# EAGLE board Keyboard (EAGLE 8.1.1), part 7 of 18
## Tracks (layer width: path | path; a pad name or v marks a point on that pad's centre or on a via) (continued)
S$6559 (continued)
  Bottom 0: 112.13,25.25 111.81,25.4
S$6560
  Bottom 0: 111.81,25.4 111.47,25.46
S$6561
  Bottom 0: 111.47,25.46 111.12,25.44
S$6562
  Bottom 0: 111.12,25.44 110.82,25.34
S$6563
  Bottom 0: 110.82,25.34 111.79,26.32
S$6564
  Bottom 0: 111.79,26.32 111.85,26.38
S$6565
  Bottom 0: 111.85,26.38 111.9,26.46
S$6566
  Bottom 0: 111.9,26.46 111.94,26.54
S$6567
  Bottom 0: 111.94,26.54 111.96,26.63
S$6568
  Bottom 0: 111.96,26.63 111.96,26.72
S$6569
  Bottom 0: 111.96,26.72 111.96,33.9
S$6570
  Bottom 0: 111.96,33.9 112.2,34.07
S$6571
  Bottom 0: 112.2,34.07 112.41,34.32
S$6572
  Bottom 0: 112.41,34.32 112.54,34.62
S$6573
  Bottom 0: 112.54,34.62 112.58,34.94
S$6574
  Bottom 0: 112.58,34.94 112.54,35.26
S$6575
  Bottom 0: 112.54,35.26 112.41,35.56
S$6576
  Bottom 0: 112.41,35.56 112.2,35.82
S$6577
  Bottom 0: 112.2,35.82 112.03,35.94
S$6578
  Bottom 0: 112.03,35.94 112.63,35.94
S$6579
  Bottom 0: 112.63,35.94 112.7,35.94
S$6580
  Bottom 0: 112.7,35.94 112.76,35.96
S$6581
  Bottom 0: 112.76,35.96 112.82,35.98
S$6582
  Bottom 0: 112.82,35.98 112.88,36.02
S$6583
  Bottom 0: 112.88,36.02 112.94,36.06
S$6584
  Bottom 0: 112.94,36.06 117.28,40.4
S$6585
  Bottom 0: 117.28,40.4 117.32,40.46
S$6586
  Bottom 0: 117.32,40.46 117.36,40.52
S$6587
  Bottom 0: 117.36,40.52 117.39,40.58
S$6588
  Bottom 0: 117.39,40.58 117.4,40.65
S$6589
  Bottom 0: 117.4,40.65 117.41,40.72
S$6590
  Bottom 0: 117.41,40.72 117.41,41.83
S$6591
  Bottom 0: 117.41,41.83 122.58,47
S$6592
  Bottom 0: 122.58,47 122.63,47.05
S$6593
  Bottom 0: 122.63,47.05 122.67,47.11
S$6594
  Bottom 0: 122.67,47.11 122.69,47.17
S$6595
  Bottom 0: 122.69,47.17 122.71,47.24
S$6596
  Bottom 0: 122.71,47.24 122.72,47.31
S$6597
  Bottom 0: 122.72,47.31 122.72,56.03
S$6598
  Bottom 0: 122.72,56.03 122.71,56.1
S$6599
  Bottom 0: 122.71,56.1 122.69,56.17
S$6600
  Bottom 0: 122.69,56.17 122.67,56.23
S$6601
  Bottom 0: 122.67,56.23 122.63,56.29
S$6602
  Bottom 0: 122.63,56.29 122.59,56.34
S$6603
  Bottom 0: 122.59,56.34 117.39,61.54
S$6604
  Bottom 0: 117.39,61.54 117.49,61.82
S$6605
  Bottom 0: 117.49,61.82 117.54,62.17
S$6606
  Bottom 0: 117.54,62.17 117.49,62.51
S$6607
  Bottom 0: 117.49,62.51 117.37,62.84
S$6608
  Bottom 0: 117.37,62.84 117.16,63.12
S$6609
  Bottom 0: 117.16,63.12 116.89,63.34
S$6610
  Bottom 0: 116.89,63.34 116.58,63.49
S$6611
  Bottom 0: 116.58,63.49 116.58,64.42
S$6612
  Bottom 0: 116.58,64.42 116.58,64.49
S$6613
  Bottom 0: 116.58,64.49 116.56,64.56
S$6614
  Bottom 0: 116.56,64.56 116.53,64.62
S$6615
  Bottom 0: 116.53,64.62 116.5,64.68
S$6616
  Bottom 0: 116.5,64.68 116.45,64.74
S$6617
  Bottom 0: 116.45,64.74 113.01,68.18
S$6618
  Bottom 0: 113.01,68.18 112.96,68.21
S$6619
  Bottom 0: 112.96,68.21 112.89,68.26
S$6620
  Bottom 0: 112.89,68.26 112.83,68.28
S$6621
  Bottom 0: 112.83,68.28 112.77,68.3
S$6622
  Bottom 0: 112.77,68.3 112.7,68.3
S$6623
  Bottom 0: 112.7,68.3 110.8,68.3
S$6624
  Bottom 0: 110.8,68.3 110.46,68.64
S$6625
  Bottom 0: 110.46,68.64 111.95,68.64
S$6626
  Bottom 0: 111.95,68.64 112.02,68.65
S$6627
  Bottom 0: 112.02,68.65 112.1,68.69
S$6628
  Bottom 0: 112.1,68.69 112.15,68.75
S$6629
  Bottom 0: 112.15,68.75 112.19,68.82
S$6630
  Bottom 0: 112.19,68.82 112.2,68.9
S$6631
  Bottom 0: 112.2,68.9 112.2,70.67
S$6632
  Bottom 0: 112.2,70.67 112.19,70.75
S$6633
  Bottom 0: 112.19,70.75 112.15,70.82
S$6634
  Bottom 0: 112.15,70.82 112.1,70.88
S$6635
  Bottom 0: 112.1,70.88 112.02,70.92
S$6636
  Bottom 0: 112.02,70.92 111.95,70.93
S$6637
  Bottom 0: 111.95,70.93 111.5,70.93
S$6638
  Bottom 0: 111.5,70.93 111.5,71.06
S$6639
  Bottom 0: 111.5,71.06 111.44,71.28
S$6640
  Bottom 0: 111.44,71.28 111.28,71.44
S$6641
  Bottom 0: 111.28,71.44 111.06,71.5
S$6642
  Bottom 0: 111.06,71.5 110.71,71.5
S$6643
  Bottom 0: 110.71,71.5 109.62,72.58
S$6644
  Bottom 0: 109.62,72.58 109.68,72.72
S$6645
  Bottom 0: 109.68,72.72 109.72,73.04
S$6646
  Bottom 0: 109.72,73.04 109.68,73.36
S$6647
  Bottom 0: 109.68,73.36 109.55,73.66
S$6648
  Bottom 0: 109.55,73.66 109.34,73.92
S$6649
  Bottom 0: 109.34,73.92 109.08,74.11
S$6650
  Bottom 0: 109.08,74.11 108.78,74.21
S$6651
  Bottom 0: 108.78,74.21 108.45,74.23
S$6652
  Bottom 0: 108.45,74.23 108.13,74.17
S$6653
  Bottom 0: 108.13,74.17 107.84,74.02
S$6654
  Bottom 0: 107.84,74.02 107.61,73.8
S$6655
  Bottom 0: 107.61,73.8 107.43,73.52
S$6656
  Bottom 0: 107.43,73.52 107.35,73.2
S$6657
  Bottom 0: 107.35,73.2 107.35,72.88
S$6658
  Bottom 0: 107.35,72.88 107.43,72.56
S$6659
  Bottom 0: 107.43,72.56 107.61,72.29
S$6660
  Bottom 0: 107.61,72.29 107.84,72.07
S$6661
  Bottom 0: 107.84,72.07 108.13,71.92
S$6662
  Bottom 0: 108.13,71.92 108.45,71.85
S$6663
  Bottom 0: 108.45,71.85 108.78,71.87
S$6664
  Bottom 0: 108.78,71.87 109,71.95
S$6665
  Bottom 0: 109,71.95 110.06,70.9
S$6666
  Bottom 0: 110.06,70.9 110.02,70.88
S$6667
  Bottom 0: 110.02,70.88 109.97,70.82
S$6668
  Bottom 0: 109.97,70.82 109.93,70.75
S$6669
  Bottom 0: 109.93,70.75 109.92,70.67
S$6670
  Bottom 0: 109.92,70.67 109.92,69.19
S$6671
  Bottom 0: 109.92,69.19 106.29,72.82
S$6672
  Bottom 0: 106.29,72.82 106.33,73.03
S$6673
  Bottom 0: 106.33,73.03 106.28,73.28
S$6674
  Bottom 0: 106.28,73.28 106.15,73.49
S$6675
  Bottom 0: 106.15,73.49 105.95,73.64
S$6676
  Bottom 0: 105.95,73.64 105.72,73.7
S$6677
  Bottom 0: 105.72,73.7 106.29,74.28
S$6678
  Bottom 0: 106.29,74.28 106.55,74.23
S$6679
  Bottom 0: 106.55,74.23 106.87,74.24
S$6680
  Bottom 0: 106.87,74.24 107.17,74.35
S$6681
  Bottom 0: 107.17,74.35 107.44,74.54
S$6682
  Bottom 0: 107.44,74.54 107.64,74.8
S$6683
  Bottom 0: 107.64,74.8 107.77,75.09
S$6684
  Bottom 0: 107.77,75.09 107.82,75.42
S$6685
  Bottom 0: 107.82,75.42 107.77,75.73
S$6686
  Bottom 0: 107.77,75.73 107.64,76.03
S$6687
  Bottom 0: 107.64,76.03 107.44,76.29
S$6688
  Bottom 0: 107.44,76.29 108.3,76.29
S$6689
  Bottom 0: 108.3,76.29 113.67,70.92
S$6690
  Bottom 0: 113.67,70.92 113.44,70.92
S$6691
  Bottom 0: 113.44,70.92 113.13,70.83
S$6692
  Bottom 0: 113.13,70.83 112.85,70.65
S$6693
  Bottom 0: 112.85,70.65 112.64,70.41
S$6694
  Bottom 0: 112.64,70.41 112.5,70.11
S$6695
  Bottom 0: 112.5,70.11 112.46,69.79
S$6696
  Bottom 0: 112.46,69.79 112.5,69.47
S$6697
  Bottom 0: 112.5,69.47 112.64,69.16
S$6698
  Bottom 0: 112.64,69.16 112.85,68.92
S$6699
  Bottom 0: 112.85,68.92 113.13,68.75
S$6700
  Bottom 0: 113.13,68.75 113.44,68.65
S$6701
  Bottom 0: 113.44,68.65 113.76,68.65
S$6702
  Bottom 0: 113.76,68.65 114.07,68.75
S$6703
  Bottom 0: 114.07,68.75 114.35,68.92
S$6704
  Bottom 0: 114.35,68.92 114.56,69.16
S$6705
  Bottom 0: 114.56,69.16 114.7,69.47
S$6706
  Bottom 0: 114.7,69.47 114.75,69.79
S$6707
  Bottom 0: 114.75,69.79 114.73,69.85
S$6708
  Bottom 0: 114.73,69.85 123.81,60.77
S$6709
  Bottom 0: 123.81,60.77 123.81,41.6
S$6710
  Bottom 0: 123.81,41.6 113.64,31.45
S$6711
  Bottom 0: 113.64,31.45 113.61,31.39
S$6712
  Bottom 0: 113.61,31.39 113.57,31.33
S$6713
  Bottom 0: 113.57,31.33 113.54,31.27
S$6714
  Bottom 0: 113.54,31.27 113.53,31.2
S$6715
  Bottom 0: 113.53,31.2 113.52,31.13
S$6716
  Bottom 0: 113.52,31.13 113.52,23.41
S$6717
  Bottom 0: 113.52,23.41 113.38,23.26
S$6718
  Bottom 0: 113.38,23.26 113.29,23.02
S$6719
  Bottom 0: 113.29,23.02 113.29,22.77
S$6720
  Bottom 0: 113.29,22.77 113.38,22.54
S$6721
  Bottom 0: 113.38,22.54 113.55,22.35
S$6722
  Bottom 0: 113.55,22.35 113.77,22.24
S$6723
  Bottom 0: 113.77,22.24 114.02,22.22
S$6724
  Bottom 0: 114.02,22.22 114.27,22.28
S$6725
  Bottom 0: 114.27,22.28 114.47,22.44
S$6726
  Bottom 0: 114.47,22.44 114.6,22.65
S$6727
  Bottom 0: 114.6,22.65 114.65,22.9
S$6728
  Bottom 0: 114.65,22.9 114.6,23.15
S$6729
  Bottom 0: 114.6,23.15 114.47,23.36
S$6730
  Bottom 0: 114.47,23.36 114.4,23.41
S$6731
  Bottom 0: 114.4,23.41 114.4,30.95
S$6732
  Bottom 0: 114.4,30.95 124.56,41.1
S$6733
  Bottom 0: 124.56,41.1 124.61,41.16
S$6734
  Bottom 0: 124.61,41.16 124.64,41.22
S$6735
  Bottom 0: 124.64,41.22 124.67,41.28
S$6736
  Bottom 0: 124.67,41.28 124.69,41.35
S$6737
  Bottom 0: 124.69,41.35 124.69,41.42
S$6738
  Bottom 0: 124.69,41.42 124.69,57.56
S$6739
  Bottom 0: 124.69,57.56 131.03,57.56
S$6740
  Bottom 0: 131.03,57.56 131.1,57.56
S$6741
  Bottom 0: 131.1,57.56 131.16,57.58
S$6742
  Bottom 0: 131.16,57.58 131.22,57.6
S$6743
  Bottom 0: 131.22,57.6 131.28,57.65
S$6744
  Bottom 0: 131.28,57.65 131.34,57.69
S$6745
  Bottom 0: 131.34,57.69 134.57,60.92
S$6746
  Bottom 0: 134.57,60.92 134.6,60.9
S$6747
  Bottom 0: 134.6,60.9 134.93,60.8
S$6748
  Bottom 0: 134.93,60.8 135.28,60.77
S$6749
  Bottom 0: 135.28,60.77 135.62,60.84
S$6750
  Bottom 0: 135.62,60.84 135.94,60.99
S$6751
  Bottom 0: 135.94,60.99 136.21,61.21
S$6752
  Bottom 0: 136.21,61.21 136.42,61.5
S$6753
  Bottom 0: 136.42,61.5 136.54,61.82
S$6754
  Bottom 0: 136.54,61.82 136.59,62.17
S$6755
  Bottom 0: 136.59,62.17 136.54,62.51
S$6756
  Bottom 0: 136.54,62.51 136.42,62.84
S$6757
  Bottom 0: 136.42,62.84 136.21,63.12
S$6758
  Bottom 0: 136.21,63.12 135.94,63.34
S$6759
  Bottom 0: 135.94,63.34 135.62,63.5
S$6760
  Bottom 0: 135.62,63.5 135.28,63.56
S$6761
  Bottom 0: 135.28,63.56 134.93,63.54
S$6762
  Bottom 0: 134.93,63.54 134.6,63.43
S$6763
  Bottom 0: 134.6,63.43 134.3,63.24
S$6764
  Bottom 0: 134.3,63.24 134.06,62.99
S$6765
  Bottom 0: 134.06,62.99 133.89,62.68
S$6766
  Bottom 0: 133.89,62.68 133.81,62.34
S$6767
  Bottom 0: 133.81,62.34 133.81,61.99
S$6768
  Bottom 0: 133.81,61.99 133.89,61.65
S$6769
  Bottom 0: 133.89,61.65 133.95,61.55
S$6770
  Bottom 0: 133.95,61.55 130.84,58.44
S$6771
  Bottom 0: 130.84,58.44 129.58,58.44
S$6772
  Bottom 0: 129.58,58.44 129.59,58.45
S$6773
  Bottom 0: 129.59,58.45 129.86,58.67
S$6774
  Bottom 0: 129.86,58.67 130.07,58.96
S$6775
  Bottom 0: 130.07,58.96 130.19,59.28
S$6776
  Bottom 0: 130.19,59.28 130.24,59.63
S$6777
  Bottom 0: 130.24,59.63 130.19,59.97
S$6778
  Bottom 0: 130.19,59.97 130.07,60.3
S$6779
  Bottom 0: 130.07,60.3 129.86,60.58
S$6780
  Bottom 0: 129.86,60.58 129.59,60.8
S$6781
  Bottom 0: 129.59,60.8 129.27,60.96
S$6782
  Bottom 0: 129.27,60.96 128.93,61.02
S$6783
  Bottom 0: 128.93,61.02 128.58,61
S$6784
  Bottom 0: 128.58,61 128.25,60.89
S$6785
  Bottom 0: 128.25,60.89 127.95,60.7
S$6786
  Bottom 0: 127.95,60.7 127.71,60.45
S$6787
  Bottom 0: 127.71,60.45 127.54,60.14
S$6788
  Bottom 0: 127.54,60.14 127.45,59.8
S$6789
  Bottom 0: 127.45,59.8 127.45,59.45
S$6790
  Bottom 0: 127.45,59.45 127.54,59.11
S$6791
  Bottom 0: 127.54,59.11 127.71,58.8
S$6792
  Bottom 0: 127.71,58.8 127.95,58.55
S$6793
  Bottom 0: 127.95,58.55 128.12,58.44
S$6794
  Bottom 0: 128.12,58.44 124.69,58.44
S$6795
  Bottom 0: 124.69,58.44 124.69,60.96
S$6796
  Bottom 0: 124.69,60.96 124.69,61.03
S$6797
  Bottom 0: 124.69,61.03 124.67,61.1
S$6798
  Bottom 0: 124.67,61.1 124.64,61.16
S$6799
  Bottom 0: 124.64,61.16 124.61,61.22
S$6800
  Bottom 0: 124.61,61.22 124.56,61.28
S$6801
  Bottom 0: 124.56,61.28 108.8,77.05
S$6802
  Bottom 0: 108.8,77.05 108.69,77.13
S$6803
  Bottom 0: 108.69,77.13 108.62,77.15
S$6804
  Bottom 0: 108.62,77.15 108.56,77.17
S$6805
  Bottom 0: 108.56,77.17 108.49,77.17
S$6806
  Bottom 0: 108.49,77.17 104.84,77.17
S$6807
  Bottom 0: 104.84,77.17 104.77,77.17
S$6808
  Bottom 0: 104.77,77.17 104.71,77.15
S$6809
  Bottom 0: 104.71,77.15 104.64,77.12
S$6810
  Bottom 0: 104.64,77.12 104.58,77.09
S$6811
  Bottom 0: 104.58,77.09 104.53,77.04
S$6812
  Bottom 0: 104.53,77.04 102.04,74.55
S$6813
  Bottom 0: 102.04,74.55 99.83,74.55
S$6814
  Bottom 0: 99.83,74.55 100.03,74.8
S$6815
  Bottom 0: 100.03,74.8 100.15,75.09
S$6816
  Bottom 0: 100.15,75.09 100.2,75.42
S$6817
  Bottom 0: 100.2,75.42 100.15,75.73
S$6818
  Bottom 0: 100.15,75.73 100.03,76.03
S$6819
  Bottom 0: 100.03,76.03 99.82,76.29
S$6820
  Bottom 0: 99.82,76.29 99.56,76.48
S$6821
  Bottom 0: 99.56,76.48 99.25,76.58
S$6822
  Bottom 0: 99.25,76.58 98.95,76.6
S$6823
  Bottom 0: 98.95,76.6 98.95,78.22
S$6824
  Bottom 0: 98.95,78.22 98.97,78.16
S$6825
  Bottom 0: 98.97,78.16 99.14,77.85
S$6826
  Bottom 0: 99.14,77.85 99.38,77.6
S$6827
  Bottom 0: 99.38,77.6 99.67,77.41
S$6828
  Bottom 0: 99.67,77.41 100,77.31
S$6829
  Bottom 0: 100,77.31 100.35,77.28
S$6830
  Bottom 0: 100.35,77.28 100.7,77.35
S$6831
  Bottom 0: 100.7,77.35 101.01,77.5
S$6832
  Bottom 0: 101.01,77.5 101.28,77.72
S$6833
  Bottom 0: 101.28,77.72 101.49,78.01
S$6834
  Bottom 0: 101.49,78.01 101.62,78.33
S$6835
  Bottom 0: 101.62,78.33 101.66,78.68
S$6836
  Bottom 0: 101.66,78.68 101.62,79.02
S$6837
  Bottom 0: 101.62,79.02 101.49,79.35
S$6838
  Bottom 0: 101.49,79.35 101.28,79.63
S$6839
  Bottom 0: 101.28,79.63 101.01,79.86
S$6840
  Bottom 0: 101.01,79.86 100.7,80.01
S$6841
  Bottom 0: 100.7,80.01 100.35,80.07
S$6842
  Bottom 0: 100.35,80.07 100,80.05
S$6843
  Bottom 0: 100,80.05 99.67,79.94
S$6844
  Bottom 0: 99.67,79.94 99.38,79.75
S$6845
  Bottom 0: 99.38,79.75 99.14,79.5
S$6846
  Bottom 0: 99.14,79.5 98.97,79.19
S$6847
  Bottom 0: 98.97,79.19 98.95,79.13
S$6848
  Bottom 0: 98.95,79.13 98.95,84.36
S$6849
  Bottom 0: 98.95,84.36 101.85,87.25
S$6850
  Bottom 0: 101.85,87.25 101.88,87.31
S$6851
  Bottom 0: 101.88,87.31 101.92,87.35
S$6852
  Bottom 0: 101.92,87.35 101.93,87.39
S$6853
  Bottom 0: 101.93,87.39 101.96,87.45
S$6854
  Bottom 0: 101.96,87.45 101.96,87.51
S$6855
  Bottom 0: 101.96,87.51 101.98,87.57
S$6856
  Bottom 0: 101.98,87.57 101.98,87.69
S$6857
  Bottom 0: 101.98,87.69 102.42,87.69
S$6858
  Bottom 0: 102.42,87.69 102.5,87.7
S$6859
  Bottom 0: 102.5,87.7 102.57,87.74
S$6860
  Bottom 0: 102.57,87.74 102.63,87.8
S$6861
  Bottom 0: 102.63,87.8 102.67,87.87
S$6862
  Bottom 0: 102.67,87.87 102.68,87.95
S$6863
  Bottom 0: 102.68,87.95 102.68,89.65
S$6864
  Bottom 0: 102.68,89.65 103.29,89.65
S$6865
  Bottom 0: 103.29,89.65 103.12,89.46
S$6866
  Bottom 0: 103.12,89.46 102.98,89.16
S$6867
  Bottom 0: 102.98,89.16 102.93,88.84
S$6868
  Bottom 0: 102.93,88.84 102.98,88.52
S$6869
  Bottom 0: 102.98,88.52 103.12,88.22
S$6870
  Bottom 0: 103.12,88.22 103.33,87.97
S$6871
  Bottom 0: 103.33,87.97 103.6,87.8
S$6872
  Bottom 0: 103.6,87.8 103.91,87.7
S$6873
  Bottom 0: 103.91,87.7 104.24,87.7
S$6874
  Bottom 0: 104.24,87.7 104.55,87.8
S$6875
  Bottom 0: 104.55,87.8 104.82,87.97
S$6876
  Bottom 0: 104.82,87.97 105.04,88.22
S$6877
  Bottom 0: 105.04,88.22 105.17,88.52
S$6878
  Bottom 0: 105.17,88.52 105.22,88.84
S$6879
  Bottom 0: 105.22,88.84 105.17,89.16
S$6880
  Bottom 0: 105.17,89.16 105.04,89.46
S$6881
  Bottom 0: 105.04,89.46 104.86,89.65
S$6882
  Bottom 0: 104.86,89.65 119.44,89.65
S$6883
  Bottom 0: 119.44,89.65 119.44,87.95
S$6884
  Bottom 0: 119.44,87.95 119.45,87.87
S$6885
  Bottom 0: 119.45,87.87 119.49,87.8
S$6886
  Bottom 0: 119.49,87.8 119.55,87.74
S$6887
  Bottom 0: 119.55,87.74 119.62,87.7
S$6888
  Bottom 0: 119.62,87.7 119.7,87.69
S$6889
  Bottom 0: 119.7,87.69 120.09,87.69
S$6890
  Bottom 0: 120.09,87.69 117.43,85.04
S$6891
  Bottom 0: 117.43,85.04 117.39,84.99
S$6892
  Bottom 0: 117.39,84.99 117.35,84.93
S$6893
  Bottom 0: 117.35,84.93 117.32,84.86
S$6894
  Bottom 0: 117.32,84.86 117.31,84.8
S$6895
  Bottom 0: 117.31,84.8 117.3,84.73
S$6896
  Bottom 0: 117.3,84.73 117.3,76.33
S$6897
  Bottom 0: 117.3,76.33 117.13,76.17
S$6898
  Bottom 0: 117.13,76.17 116.96,75.89
S$6899
  Bottom 0: 116.96,75.89 116.87,75.58
S$6900
  Bottom 0: 116.87,75.58 116.87,75.26
S$6901
  Bottom 0: 116.87,75.26 116.96,74.94
S$6902
  Bottom 0: 116.96,74.94 117.03,74.83
S$6903
  Bottom 0: 117.03,74.83 114.25,77.61
S$6904
  Bottom 0: 114.25,77.61 114.2,77.64
S$6905
  Bottom 0: 114.2,77.64 114.14,77.69
S$6906
  Bottom 0: 114.14,77.69 114.07,77.71
S$6907
  Bottom 0: 114.07,77.71 114.01,77.73
S$6908
  Bottom 0: 114.01,77.73 113.94,77.73
S$6909
  Bottom 0: 113.94,77.73 110.73,77.73
S$6910
  Bottom 0: 110.73,77.73 107.86,80.6
S$6911
  Bottom 0: 107.86,80.6 107.97,80.87
S$6912
  Bottom 0: 107.97,80.87 108.01,81.22
S$6913
  Bottom 0: 108.01,81.22 107.97,81.56
S$6914
  Bottom 0: 107.97,81.56 107.84,81.89
S$6915
  Bottom 0: 107.84,81.89 107.63,82.17
S$6916
  Bottom 0: 107.63,82.17 107.36,82.39
S$6917
  Bottom 0: 107.36,82.39 107.05,82.55
S$6918
  Bottom 0: 107.05,82.55 106.7,82.61
S$6919
  Bottom 0: 106.7,82.61 106.35,82.59
S$6920
  Bottom 0: 106.35,82.59 106.02,82.48
S$6921
  Bottom 0: 106.02,82.48 105.73,82.29
S$6922
  Bottom 0: 105.73,82.29 105.49,82.04
S$6923
  Bottom 0: 105.49,82.04 105.32,81.73
S$6924
  Bottom 0: 105.32,81.73 105.23,81.39
S$6925
  Bottom 0: 105.23,81.39 105.23,81.04
S$6926
  Bottom 0: 105.23,81.04 105.32,80.7
S$6927
  Bottom 0: 105.32,80.7 105.49,80.39
S$6928
  Bottom 0: 105.49,80.39 105.73,80.14
S$6929
  Bottom 0: 105.73,80.14 106.02,79.95
S$6930
  Bottom 0: 106.02,79.95 106.35,79.84
S$6931
  Bottom 0: 106.35,79.84 106.7,79.83
S$6932
  Bottom 0: 106.7,79.83 107.05,79.89
S$6933
  Bottom 0: 107.05,79.89 107.23,79.97
S$6934
  Bottom 0: 107.23,79.97 110.23,76.97
S$6935
  Bottom 0: 110.23,76.97 110.28,76.93
S$6936
  Bottom 0: 110.28,76.93 110.34,76.89
S$6937
  Bottom 0: 110.34,76.89 110.4,76.87
S$6938
  Bottom 0: 110.4,76.87 110.47,76.85
S$6939
  Bottom 0: 110.47,76.85 110.54,76.85
S$6940
  Bottom 0: 110.54,76.85 113.75,76.85
S$6941
  Bottom 0: 113.75,76.85 116.39,74.21
S$6942
  Bottom 0: 116.39,74.21 116.07,74.23
S$6943
  Bottom 0: 116.07,74.23 115.75,74.17
S$6944
  Bottom 0: 115.75,74.17 115.46,74.02
S$6945
  Bottom 0: 115.46,74.02 115.23,73.8
S$6946
  Bottom 0: 115.23,73.8 115.05,73.52
S$6947
  Bottom 0: 115.05,73.52 114.97,73.2
S$6948
  Bottom 0: 114.97,73.2 114.97,72.88
S$6949
  Bottom 0: 114.97,72.88 115.05,72.56
S$6950
  Bottom 0: 115.05,72.56 115.23,72.29
S$6951
  Bottom 0: 115.23,72.29 115.46,72.07
S$6952
  Bottom 0: 115.46,72.07 115.75,71.92
S$6953
  Bottom 0: 115.75,71.92 116.07,71.85
S$6954
  Bottom 0: 116.07,71.85 116.39,71.87
S$6955
  Bottom 0: 116.39,71.87 116.7,71.98
S$6956
  Bottom 0: 116.7,71.98 116.96,72.17
S$6957
  Bottom 0: 116.96,72.17 117.17,72.42
S$6958
  Bottom 0: 117.17,72.42 117.19,72.47
S$6959
  Bottom 0: 117.19,72.47 123.36,72.47
S$6960
  Bottom 0: 123.36,72.47 123.45,72.48
S$6961
  Bottom 0: 123.45,72.48 123.54,72.5
S$6962
  Bottom 0: 123.54,72.5 123.62,72.53
S$6963
  Bottom 0: 123.62,72.53 123.7,72.58
S$6964
  Bottom 0: 123.7,72.58 123.77,72.64
S$6965
  Bottom 0: 123.77,72.64 125.4,74.27
S$6966
  Bottom 0: 125.4,74.27 125.59,74.23
S$6967
  Bottom 0: 125.59,74.23 125.92,74.25
S$6968
  Bottom 0: 125.92,74.25 126.22,74.36
S$6969
  Bottom 0: 126.22,74.36 126.49,74.55
S$6970
  Bottom 0: 126.49,74.55 126.69,74.78
S$6971
  Bottom 0: 126.69,74.78 132.66,74.78
S$6972
  Bottom 0: 132.66,74.78 134.07,73.38
S$6973
  Bottom 0: 134.07,73.38 134.02,73.2
S$6974
  Bottom 0: 134.02,73.2 134.02,72.88
S$6975
  Bottom 0: 134.02,72.88 134.11,72.56
S$6976
  Bottom 0: 134.11,72.56 134.28,72.29
S$6977
  Bottom 0: 134.28,72.29 134.52,72.07
S$6978
  Bottom 0: 134.52,72.07 134.81,71.92
S$6979
  Bottom 0: 134.81,71.92 135.12,71.85
S$6980
  Bottom 0: 135.12,71.85 135.45,71.87
S$6981
  Bottom 0: 135.45,71.87 135.75,71.98
S$6982
  Bottom 0: 135.75,71.98 136.02,72.17
S$6983
  Bottom 0: 136.02,72.17 136.23,72.42
S$6984
  Bottom 0: 136.23,72.42 136.35,72.72
S$6985
  Bottom 0: 136.35,72.72 136.4,73.04
S$6986
  Bottom 0: 136.4,73.04 136.35,73.36
S$6987
  Bottom 0: 136.35,73.36 136.28,73.54
S$6988
  Bottom 0: 136.28,73.54 145.33,73.54
S$6989
  Bottom 0: 145.33,73.54 145.4,73.54
S$6990
  Bottom 0: 145.4,73.54 145.46,73.56
S$6991
  Bottom 0: 145.46,73.56 145.52,73.59
S$6992
  Bottom 0: 145.52,73.59 145.58,73.63
S$6993
  Bottom 0: 145.58,73.63 145.63,73.66
S$6994
  Bottom 0: 145.63,73.66 145.54,73.52
S$6995
  Bottom 0: 145.54,73.52 145.45,73.2
S$6996
  Bottom 0: 145.45,73.2 145.45,72.88
S$6997
  Bottom 0: 145.45,72.88 145.54,72.56
S$6998
  Bottom 0: 145.54,72.56 145.71,72.29
S$6999
  Bottom 0: 145.71,72.29 145.95,72.07
S$7000
  Bottom 0: 145.95,72.07 146.24,71.92
S$7001
  Bottom 0: 146.24,71.92 146.56,71.85
S$7002
  Bottom 0: 146.56,71.85 146.88,71.87
S$7003
  Bottom 0: 146.88,71.87 147.1,71.95
S$7004
  Bottom 0: 147.1,71.95 148.16,70.89
S$7005
  Bottom 0: 148.16,70.89 148.12,70.88
S$7006
  Bottom 0: 148.12,70.88 148.07,70.82
S$7007
  Bottom 0: 148.07,70.82 148.03,70.75
S$7008
  Bottom 0: 148.03,70.75 148.02,70.67
S$7009
  Bottom 0: 148.02,70.67 148.02,68.9
S$7010
  Bottom 0: 148.02,68.9 148.03,68.82
S$7011
  Bottom 0: 148.03,68.82 148.07,68.75
S$7012
  Bottom 0: 148.07,68.75 148.12,68.69
S$7013
  Bottom 0: 148.12,68.69 148.2,68.65
S$7014
  Bottom 0: 148.2,68.65 148.27,68.64
S$7015
  Bottom 0: 148.27,68.64 149.76,68.64
S$7016
  Bottom 0: 149.76,68.64 146.68,65.57
S$7017
  Bottom 0: 146.68,65.57 141.78,70.46
S$7018
  Bottom 0: 141.78,70.46 141.72,70.52
S$7019
  Bottom 0: 141.72,70.52 141.64,70.56
S$7020
  Bottom 0: 141.64,70.56 141.56,70.6
S$7021
  Bottom 0: 141.56,70.6 141.47,70.62
S$7022
  Bottom 0: 141.47,70.62 141.38,70.62
S$7023
  Bottom 0: 141.38,70.62 133.42,70.62
S$7024
  Bottom 0: 133.42,70.62 133.4,70.65
S$7025
  Bottom 0: 133.4,70.65 133.12,70.83
S$7026
  Bottom 0: 133.12,70.83 132.81,70.92
S$7027
  Bottom 0: 132.81,70.92 132.49,70.92
S$7028
  Bottom 0: 132.49,70.92 132.18,70.83
S$7029
  Bottom 0: 132.18,70.83 131.9,70.65
S$7030
  Bottom 0: 131.9,70.65 131.69,70.41
S$7031
  Bottom 0: 131.69,70.41 131.55,70.11
S$7032
  Bottom 0: 131.55,70.11 131.51,69.79
S$7033
  Bottom 0: 131.51,69.79 131.55,69.47
S$7034
  Bottom 0: 131.55,69.47 131.69,69.16
S$7035
  Bottom 0: 131.69,69.16 131.9,68.92
S$7036
  Bottom 0: 131.9,68.92 132.02,68.85
S$7037
  Bottom 0: 132.02,68.85 131.25,68.85
S$7038
  Bottom 0: 131.25,68.85 131.25,68.9
S$7039
  Bottom 0: 131.25,68.9 131.25,70.67
S$7040
  Bottom 0: 131.25,70.67 131.24,70.75
S$7041
  Bottom 0: 131.24,70.75 131.2,70.82
S$7042
  Bottom 0: 131.2,70.82 131.15,70.88
S$7043
  Bottom 0: 131.15,70.88 131.07,70.92
S$7044
  Bottom 0: 131.07,70.92 131,70.93
S$7045
  Bottom 0: 131,70.93 130.55,70.93
S$7046
  Bottom 0: 130.55,70.93 130.55,71.06
S$7047
  Bottom 0: 130.55,71.06 130.49,71.28
S$7048
  Bottom 0: 130.49,71.28 130.33,71.44
S$7049
  Bottom 0: 130.33,71.44 130.11,71.5
S$7050
  Bottom 0: 130.11,71.5 129.76,71.5
S$7051
  Bottom 0: 129.76,71.5 128.67,72.59
S$7052
  Bottom 0: 128.67,72.59 128.74,72.72
S$7053
  Bottom 0: 128.74,72.72 128.78,73.04
S$7054
  Bottom 0: 128.78,73.04 128.74,73.36
S$7055
  Bottom 0: 128.74,73.36 128.61,73.66
S$7056
  Bottom 0: 128.61,73.66 128.4,73.92
S$7057
  Bottom 0: 128.4,73.92 128.13,74.11
S$7058
  Bottom 0: 128.13,74.11 127.83,74.21
S$7059
  Bottom 0: 127.83,74.21 127.5,74.23
S$7060
  Bottom 0: 127.5,74.23 127.19,74.17
S$7061
  Bottom 0: 127.19,74.17 126.9,74.02
S$7062
  Bottom 0: 126.9,74.02 126.66,73.8
S$7063
  Bottom 0: 126.66,73.8 126.49,73.52
S$7064
  Bottom 0: 126.49,73.52 126.4,73.2
S$7065
  Bottom 0: 126.4,73.2 126.4,72.88
S$7066
  Bottom 0: 126.4,72.88 126.49,72.56
S$7067
  Bottom 0: 126.49,72.56 126.66,72.29
S$7068
  Bottom 0: 126.66,72.29 126.9,72.07
S$7069
  Bottom 0: 126.9,72.07 127.19,71.92
S$7070
  Bottom 0: 127.19,71.92 127.5,71.85
S$7071
  Bottom 0: 127.5,71.85 127.83,71.87
S$7072
  Bottom 0: 127.83,71.87 128.05,71.95
S$7073
  Bottom 0: 128.05,71.95 129.11,70.89
S$7074
  Bottom 0: 129.11,70.89 129.07,70.88
S$7075
  Bottom 0: 129.07,70.88 129.02,70.82
S$7076
  Bottom 0: 129.02,70.82 128.98,70.75
S$7077
  Bottom 0: 128.98,70.75 128.97,70.67
S$7078
  Bottom 0: 128.97,70.67 128.97,68.9
S$7079
  Bottom 0: 128.97,68.9 128.97,68.85
S$7080
  Bottom 0: 128.97,68.85 122.87,68.85
S$7081
  Bottom 0: 122.87,68.85 122.84,69.05
S$7082
  Bottom 0: 122.84,69.05 122.7,69.32
S$7083
  Bottom 0: 122.7,69.32 122.5,69.54
S$7084
  Bottom 0: 122.5,69.54 122.24,69.69
S$7085
  Bottom 0: 122.24,69.69 121.94,69.76
S$7086
  Bottom 0: 121.94,69.76 121.64,69.74
S$7087
  Bottom 0: 121.64,69.74 121.36,69.63
S$7088
  Bottom 0: 121.36,69.63 121.12,69.44
S$7089
  Bottom 0: 121.12,69.44 120.95,69.19
S$7090
  Bottom 0: 120.95,69.19 120.86,68.9
S$7091
  Bottom 0: 120.86,68.9 120.86,68.59
S$7092
  Bottom 0: 120.86,68.59 120.95,68.31
S$7093
  Bottom 0: 120.95,68.31 121.12,68.06
S$7094
  Bottom 0: 121.12,68.06 121.36,67.87
S$7095
  Bottom 0: 121.36,67.87 121.64,67.76
S$7096
  Bottom 0: 121.64,67.76 121.94,67.74
S$7097
  Bottom 0: 121.94,67.74 122.24,67.81
S$7098
  Bottom 0: 122.24,67.81 122.5,67.95
S$7099
  Bottom 0: 122.5,67.95 122.51,67.97
S$7100
  Bottom 0: 122.51,67.97 140.28,67.97
S$7101
  Bottom 0: 140.28,67.97 140.4,67.87
S$7102
  Bottom 0: 140.4,67.87 140.68,67.76
S$7103
  Bottom 0: 140.68,67.76 140.99,67.74
S$7104
  Bottom 0: 140.99,67.74 141.28,67.81
S$7105
  Bottom 0: 141.28,67.81 141.55,67.95
S$7106
  Bottom 0: 141.55,67.95 141.75,68.18
S$7107
  Bottom 0: 141.75,68.18 141.88,68.45
S$7108
  Bottom 0: 141.88,68.45 141.92,68.72
S$7109
  Bottom 0: 141.92,68.72 145.87,64.77
S$7110
  Bottom 0: 145.87,64.77 141.83,60.72
S$7111
  Bottom 0: 141.83,60.72 141.88,60.83
S$7112
  Bottom 0: 141.88,60.83 141.93,61.13
S$7113
  Bottom 0: 141.93,61.13 141.88,61.43
S$7114
  Bottom 0: 141.88,61.43 141.75,61.7
S$7115
  Bottom 0: 141.75,61.7 141.55,61.92
S$7116
  Bottom 0: 141.55,61.92 141.28,62.08
S$7117
  Bottom 0: 141.28,62.08 140.99,62.14
S$7118
  Bottom 0: 140.99,62.14 140.68,62.12
S$7119
  Bottom 0: 140.68,62.12 140.4,62.01
S$7120
  Bottom 0: 140.4,62.01 140.16,61.82
S$7121
  Bottom 0: 140.16,61.82 140,61.57
S$7122
  Bottom 0: 140,61.57 139.9,61.28
S$7123
  Bottom 0: 139.9,61.28 139.9,60.98
S$7124
  Bottom 0: 139.9,60.98 140,60.69
S$7125
  Bottom 0: 140,60.69 140.16,60.44
S$7126
  Bottom 0: 140.16,60.44 140.4,60.25
S$7127
  Bottom 0: 140.4,60.25 140.68,60.14
S$7128
  Bottom 0: 140.68,60.14 140.99,60.12
S$7129
  Bottom 0: 140.99,60.12 141.28,60.19
S$7130
  Bottom 0: 141.28,60.19 141.31,60.2
S$7131
  Bottom 0: 141.31,60.2 137.01,55.9
S$7132
  Bottom 0: 137.01,55.9 136.95,55.83
S$7133
  Bottom 0: 136.95,55.83 136.9,55.76
S$7134
  Bottom 0: 136.9,55.76 136.87,55.67
S$7135
  Bottom 0: 136.87,55.67 136.85,55.59
S$7136
  Bottom 0: 136.85,55.59 136.84,55.5
S$7137
  Bottom 0: 136.84,55.5 136.84,51.72
S$7138
  Bottom 0: 136.84,51.72 136.66,51.6
S$7139
  Bottom 0: 136.66,51.6 136.45,51.36
S$7140
  Bottom 0: 136.45,51.36 136.31,51.06
S$7141
  Bottom 0: 136.31,51.06 136.27,50.74
S$7142
  Bottom 0: 136.27,50.74 136.31,50.42
S$7143
  Bottom 0: 136.31,50.42 136.45,50.11
S$7144
  Bottom 0: 136.45,50.11 136.66,49.88
S$7145
  Bottom 0: 136.66,49.88 136.01,49.88
S$7146
  Bottom 0: 136.01,49.88 136.01,51.63
S$7147
  Bottom 0: 136.01,51.63 136,51.7
S$7148
  Bottom 0: 136,51.7 135.96,51.77
S$7149
  Bottom 0: 135.96,51.77 135.91,51.83
S$7150
  Bottom 0: 135.91,51.83 135.84,51.87
S$7151
  Bottom 0: 135.84,51.87 135.76,51.88
S$7152
  Bottom 0: 135.76,51.88 135.31,51.88
S$7153
  Bottom 0: 135.31,51.88 135.31,52.01
S$7154
  Bottom 0: 135.31,52.01 135.25,52.23
S$7155
  Bottom 0: 135.25,52.23 135.09,52.39
S$7156
  Bottom 0: 135.09,52.39 134.87,52.45
S$7157
  Bottom 0: 134.87,52.45 134.52,52.45
S$7158
  Bottom 0: 134.52,52.45 133.43,53.54
S$7159
  Bottom 0: 133.43,53.54 133.5,53.67
S$7160
  Bottom 0: 133.5,53.67 133.54,53.99
S$7161
  Bottom 0: 133.54,53.99 133.5,54.31
S$7162
  Bottom 0: 133.5,54.31 133.37,54.61
S$7163
  Bottom 0: 133.37,54.61 133.16,54.87
S$7164
  Bottom 0: 133.16,54.87 132.9,55.05
S$7165
  Bottom 0: 132.9,55.05 132.59,55.16
S$7166
  Bottom 0: 132.59,55.16 132.26,55.18
S$7167
  Bottom 0: 132.26,55.18 131.94,55.12
S$7168
  Bottom 0: 131.94,55.12 131.66,54.97
S$7169
  Bottom 0: 131.66,54.97 131.42,54.74
S$7170
  Bottom 0: 131.42,54.74 131.25,54.47
S$7171
  Bottom 0: 131.25,54.47 131.16,54.16
S$7172
  Bottom 0: 131.16,54.16 131.16,53.83
S$7173
  Bottom 0: 131.16,53.83 131.25,53.52
S$7174
  Bottom 0: 131.25,53.52 131.42,53.24
S$7175
  Bottom 0: 131.42,53.24 131.66,53.02
S$7176
  Bottom 0: 131.66,53.02 131.94,52.87
S$7177
  Bottom 0: 131.94,52.87 132.26,52.8
S$7178
  Bottom 0: 132.26,52.8 132.59,52.82
S$7179
  Bottom 0: 132.59,52.82 132.81,52.9
S$7180
  Bottom 0: 132.81,52.9 133.87,51.84
S$7181
  Bottom 0: 133.87,51.84 133.84,51.83
S$7182
  Bottom 0: 133.84,51.83 133.78,51.77
S$7183
  Bottom 0: 133.78,51.77 133.74,51.7
S$7184
  Bottom 0: 133.74,51.7 133.73,51.63
S$7185
  Bottom 0: 133.73,51.63 133.73,49.88
S$7186
  Bottom 0: 133.73,49.88 127.61,49.88
S$7187
  Bottom 0: 127.61,49.88 127.59,50
S$7188
  Bottom 0: 127.59,50 127.46,50.27
S$7189
  Bottom 0: 127.46,50.27 127.26,50.49
S$7190
  Bottom 0: 127.26,50.49 126.99,50.65
S$7191
  Bottom 0: 126.99,50.65 126.69,50.71
S$7192
  Bottom 0: 126.69,50.71 126.39,50.69
S$7193
  Bottom 0: 126.39,50.69 126.11,50.58
S$7194
  Bottom 0: 126.11,50.58 125.88,50.39
S$7195
  Bottom 0: 125.88,50.39 125.71,50.14
S$7196
  Bottom 0: 125.71,50.14 125.61,49.85
S$7197
  Bottom 0: 125.61,49.85 125.61,49.55
S$7198
  Bottom 0: 125.61,49.55 125.71,49.26
S$7199
  Bottom 0: 125.71,49.26 125.88,49.01
S$7200
  Bottom 0: 125.88,49.01 126.11,48.82
S$7201
  Bottom 0: 126.11,48.82 126.39,48.71
S$7202
  Bottom 0: 126.39,48.71 126.69,48.69
S$7203
  Bottom 0: 126.69,48.69 126.99,48.76
S$7204
  Bottom 0: 126.99,48.76 127.26,48.91
S$7205
  Bottom 0: 127.26,48.91 127.34,49
S$7206
  Bottom 0: 127.34,49 144.94,49
S$7207
  Bottom 0: 144.94,49 145.17,48.82
S$7208
  Bottom 0: 145.17,48.82 145.45,48.71
S$7209
  Bottom 0: 145.45,48.71 145.66,48.69
S$7210
  Bottom 0: 145.66,48.69 141,44.03
S$7211
  Bottom 0: 141,44.03 140.97,44.07
S$7212
  Bottom 0: 140.97,44.07 140.7,44.3
S$7213
  Bottom 0: 140.7,44.3 140.38,44.45
S$7214
  Bottom 0: 140.38,44.45 140.04,44.51
S$7215
  Bottom 0: 140.04,44.51 139.69,44.49
S$7216
  Bottom 0: 139.69,44.49 139.36,44.38
S$7217
  Bottom 0: 139.36,44.38 139.06,44.19
S$7218
  Bottom 0: 139.06,44.19 138.82,43.94
S$7219
  Bottom 0: 138.82,43.94 138.65,43.63
S$7220
  Bottom 0: 138.65,43.63 138.56,43.29
S$7221
  Bottom 0: 138.56,43.29 138.56,42.94
S$7222
  Bottom 0: 138.56,42.94 138.65,42.6
S$7223
  Bottom 0: 138.65,42.6 138.82,42.29
S$7224
  Bottom 0: 138.82,42.29 139.06,42.04
S$7225
  Bottom 0: 139.06,42.04 139.36,41.85
S$7226
  Bottom 0: 139.36,41.85 139.69,41.74
S$7227
  Bottom 0: 139.69,41.74 140.04,41.73
S$7228
  Bottom 0: 140.04,41.73 140.15,41.74
S$7229
  Bottom 0: 140.15,41.74 137.81,39.4
S$7230
  Bottom 0: 137.81,39.4 134.35,39.4
S$7231
  Bottom 0: 134.35,39.4 134.62,39.62
S$7232
  Bottom 0: 134.62,39.62 134.82,39.91
S$7233
  Bottom 0: 134.82,39.91 134.95,40.23
S$7234
  Bottom 0: 134.95,40.23 135,40.58
S$7235
  Bottom 0: 135,40.58 134.95,40.92
S$7236
  Bottom 0: 134.95,40.92 134.82,41.25
S$7237
  Bottom 0: 134.82,41.25 134.62,41.53
S$7238
  Bottom 0: 134.62,41.53 134.35,41.76
S$7239
  Bottom 0: 134.35,41.76 134.03,41.91
S$7240
  Bottom 0: 134.03,41.91 133.69,41.97
S$7241
  Bottom 0: 133.69,41.97 133.34,41.95
S$7242
  Bottom 0: 133.34,41.95 133.01,41.84
S$7243
  Bottom 0: 133.01,41.84 132.98,41.83
S$7244
  Bottom 0: 132.98,41.83 132.41,42.4
S$7245
  Bottom 0: 132.41,42.4 132.36,42.43
S$7246
  Bottom 0: 132.36,42.43 132.3,42.48
S$7247
  Bottom 0: 132.3,42.48 132.24,42.5
S$7248
  Bottom 0: 132.24,42.5 132.17,42.52
S$7249
  Bottom 0: 132.17,42.52 132.1,42.52
S$7250
  Bottom 0: 132.1,42.52 127.53,42.52
S$7251
  Bottom 0: 127.53,42.52 127.46,42.65
S$7252
  Bottom 0: 127.46,42.65 127.26,42.87
S$7253
  Bottom 0: 127.26,42.87 126.99,43.02
S$7254
  Bottom 0: 126.99,43.02 126.69,43.09
S$7255
  Bottom 0: 126.69,43.09 126.39,43.07
S$7256
  Bottom 0: 126.39,43.07 126.11,42.96
S$7257
  Bottom 0: 126.11,42.96 125.88,42.77
S$7258
  Bottom 0: 125.88,42.77 125.71,42.52
S$7259
  Bottom 0: 125.71,42.52 125.61,42.23
S$7260
  Bottom 0: 125.61,42.23 125.61,41.92
S$7261
  Bottom 0: 125.61,41.92 125.71,41.64
S$7262
  Bottom 0: 125.71,41.64 125.88,41.39
S$7263
  Bottom 0: 125.88,41.39 126.11,41.2
S$7264
  Bottom 0: 126.11,41.2 126.39,41.09
S$7265
  Bottom 0: 126.39,41.09 126.69,41.07
S$7266
  Bottom 0: 126.69,41.07 126.99,41.13
S$7267
  Bottom 0: 126.99,41.13 127.26,41.28
S$7268
  Bottom 0: 127.26,41.28 127.46,41.51
S$7269
  Bottom 0: 127.46,41.51 127.53,41.64
S$7270
  Bottom 0: 127.53,41.64 131.91,41.64
S$7271
  Bottom 0: 131.91,41.64 132.36,41.19
S$7272
  Bottom 0: 132.36,41.19 132.3,41.09
S$7273
  Bottom 0: 132.3,41.09 132.22,40.75
S$7274
  Bottom 0: 132.22,40.75 132.22,40.4
S$7275
  Bottom 0: 132.22,40.4 132.3,40.06
S$7276
  Bottom 0: 132.3,40.06 132.47,39.75
S$7277
  Bottom 0: 132.47,39.75 132.71,39.5
S$7278
  Bottom 0: 132.71,39.5 132.87,39.4
S$7279
  Bottom 0: 132.87,39.4 123.8,39.4
S$7280
  Bottom 0: 123.8,39.4 123.73,39.4
S$7281
  Bottom 0: 123.73,39.4 123.67,39.38
S$7282
  Bottom 0: 123.67,39.38 123.6,39.36
S$7283
  Bottom 0: 123.6,39.36 123.54,39.32
S$7284
  Bottom 0: 123.54,39.32 123.48,39.28
S$7285
  Bottom 0: 123.48,39.28 115.59,31.38
S$7286
  Bottom 0: 115.59,31.38 115.55,31.32
S$7287
  Bottom 0: 115.55,31.32 115.51,31.26
S$7288
  Bottom 0: 115.51,31.26 115.48,31.2
S$7289
  Bottom 0: 115.48,31.2 115.47,31.13
S$7290
  Bottom 0: 115.47,31.13 115.46,31.06
S$7291
  Bottom 0: 115.46,31.06 115.46,26.69
S$7292
  Bottom 0: 115.46,26.69 115.47,26.62
S$7293
  Bottom 0: 115.47,26.62 115.48,26.56
S$7294
  Bottom 0: 115.48,26.56 115.51,26.5
S$7295
  Bottom 0: 115.51,26.5 115.55,26.43
S$7296
  Bottom 0: 115.55,26.43 115.59,26.38
S$7297
  Bottom 0: 115.59,26.38 121.87,20.09
S$7298
  Bottom 0: 121.87,20.09 105.77,4
S$7299
  Bottom 0: 114.32,14.87 114.62,14.94
S$7300
  Bottom 0: 114.62,14.94 114.88,15.09
S$7301
  Bottom 0: 114.88,15.09 115.08,15.31
S$7302
  Bottom 0: 115.08,15.31 115.15,15.44
S$7303
  Bottom 0: 115.15,15.44 115.57,15.44
S$7304
  Bottom 0: 115.57,15.44 115.64,15.45
S$7305
  Bottom 0: 115.64,15.45 115.71,15.46
S$7306
  Bottom 0: 115.71,15.46 115.77,15.49
S$7307
  Bottom 0: 115.77,15.49 115.83,15.53
S$7308
  Bottom 0: 115.83,15.53 115.89,15.57
S$7309
  Bottom 0: 115.89,15.57 117.39,17.07
S$7310
  Bottom 0: 117.39,17.07 117.49,17.06
S$7311
  Bottom 0: 117.49,17.06 117.74,17.12
S$7312
  Bottom 0: 117.74,17.12 117.94,17.27
S$7313
  Bottom 0: 117.94,17.27 118.07,17.49
S$7314
  Bottom 0: 118.07,17.49 118.12,17.74
S$7315
  Bottom 0: 118.12,17.74 118.07,17.99
S$7316
  Bottom 0: 118.07,17.99 117.94,18.2
S$7317
  Bottom 0: 117.94,18.2 117.74,18.35
S$7318
  Bottom 0: 117.74,18.35 117.49,18.42
S$7319
  Bottom 0: 117.49,18.42 117.24,18.4
S$7320
  Bottom 0: 117.24,18.4 117.02,18.29
S$7321
  Bottom 0: 117.02,18.29 116.85,18.1
S$7322
  Bottom 0: 116.85,18.1 116.75,17.86
S$7323
  Bottom 0: 116.75,17.86 116.75,17.7
S$7324
  Bottom 0: 116.75,17.7 115.39,16.32
S$7325
  Bottom 0: 115.39,16.32 115.15,16.32
S$7326
  Bottom 0: 115.15,16.32 115.08,16.46
S$7327
  Bottom 0: 115.08,16.46 114.88,16.68
S$7328
  Bottom 0: 114.88,16.68 114.62,16.83
S$7329
  Bottom 0: 114.62,16.83 114.32,16.89
S$7330
  Bottom 0: 114.32,16.89 114.02,16.87
S$7331
  Bottom 0: 114.02,16.87 113.74,16.76
S$7332
  Bottom 0: 113.74,16.76 113.5,16.57
S$7333
  Bottom 0: 113.5,16.57 113.33,16.32
S$7334
  Bottom 0: 113.33,16.32 113.24,16.04
S$7335
  Bottom 0: 113.24,16.04 113.24,15.73
S$7336
  Bottom 0: 113.24,15.73 113.33,15.44
S$7337
  Bottom 0: 113.33,15.44 113.5,15.19
S$7338
  Bottom 0: 113.5,15.19 113.74,15
S$7339
  Bottom 0: 113.74,15 114.02,14.89
S$7340
  Bottom 0: 114.02,14.89 114.32,14.87
S$7341
  Bottom 0: 117.18,22.02 117.47,22.09
S$7342
  Bottom 0: 117.47,22.09 117.74,22.24
S$7343
  Bottom 0: 117.74,22.24 117.94,22.46
S$7344
  Bottom 0: 117.94,22.46 118.07,22.73
S$7345
  Bottom 0: 118.07,22.73 118.12,23.03
S$7346
  Bottom 0: 118.12,23.03 118.07,23.33
S$7347
  Bottom 0: 118.07,23.33 117.94,23.6
S$7348
  Bottom 0: 117.94,23.6 117.74,23.82
S$7349
  Bottom 0: 117.74,23.82 117.47,23.98
S$7350
  Bottom 0: 117.47,23.98 117.18,24.04
S$7351
  Bottom 0: 117.18,24.04 116.87,24.02
S$7352
  Bottom 0: 116.87,24.02 116.59,23.91
S$7353
  Bottom 0: 116.59,23.91 116.36,23.72
S$7354
  Bottom 0: 116.36,23.72 116.19,23.47
S$7355
  Bottom 0: 116.19,23.47 116.1,23.18
S$7356
  Bottom 0: 116.1,23.18 116.1,22.88
S$7357
  Bottom 0: 116.1,22.88 116.19,22.59
S$7358
  Bottom 0: 116.19,22.59 116.36,22.34
S$7359
  Bottom 0: 116.36,22.34 116.59,22.15
S$7360
  Bottom 0: 116.59,22.15 116.87,22.04
S$7361
  Bottom 0: 116.87,22.04 117.18,22.02
S$7362
  Bottom 0: 120.99,41.73 121.33,41.79
S$7363
  Bottom 0: 121.33,41.79 121.65,41.94
S$7364
  Bottom 0: 121.65,41.94 121.92,42.16
S$7365
  Bottom 0: 121.92,42.16 122.12,42.45
S$7366
  Bottom 0: 122.12,42.45 122.25,42.77
S$7367
  Bottom 0: 122.25,42.77 122.3,43.12
S$7368
  Bottom 0: 122.3,43.12 122.25,43.46
S$7369
  Bottom 0: 122.25,43.46 122.12,43.79
S$7370
  Bottom 0: 122.12,43.79 121.92,44.07
S$7371
  Bottom 0: 121.92,44.07 121.65,44.3
S$7372
  Bottom 0: 121.65,44.3 121.33,44.45
S$7373
  Bottom 0: 121.33,44.45 120.99,44.51
S$7374
  Bottom 0: 120.99,44.51 120.64,44.49
S$7375
  Bottom 0: 120.64,44.49 120.31,44.38
S$7376
  Bottom 0: 120.31,44.38 120.01,44.19
S$7377
  Bottom 0: 120.01,44.19 119.77,43.94
S$7378
  Bottom 0: 119.77,43.94 119.6,43.63
S$7379
  Bottom 0: 119.6,43.63 119.52,43.29
S$7380
  Bottom 0: 119.52,43.29 119.52,42.94
S$7381
  Bottom 0: 119.52,42.94 119.6,42.6
S$7382
  Bottom 0: 119.6,42.6 119.77,42.29
S$7383
  Bottom 0: 119.77,42.29 120.01,42.04
S$7384
  Bottom 0: 120.01,42.04 120.31,41.85
S$7385
  Bottom 0: 120.31,41.85 120.64,41.74
S$7386
  Bottom 0: 120.64,41.74 120.99,41.73
S$7387
  Bottom 0: 136.14,43.37 136.59,43.42
S$7388
  Bottom 0: 136.59,43.42 137.01,43.54
S$7389
  Bottom 0: 137.01,43.54 137.41,43.76
S$7390
  Bottom 0: 137.41,43.76 137.76,44.04
S$7391
  Bottom 0: 137.76,44.04 138.04,44.39
S$7392
  Bottom 0: 138.04,44.39 138.25,44.78
S$7393
  Bottom 0: 138.25,44.78 138.38,45.21
S$7394
  Bottom 0: 138.38,45.21 138.43,45.66
S$7395
  Bottom 0: 138.43,45.66 138.38,46.1
S$7396
  Bottom 0: 138.38,46.1 138.25,46.53
S$7397
  Bottom 0: 138.25,46.53 138.04,46.93
S$7398
  Bottom 0: 138.04,46.93 137.76,47.27
S$7399
  Bottom 0: 137.76,47.27 137.41,47.56
S$7400
  Bottom 0: 137.41,47.56 137.01,47.77
S$7401
  Bottom 0: 137.01,47.77 136.59,47.89
S$7402
  Bottom 0: 136.59,47.89 136.14,47.94
S$7403
  Bottom 0: 136.14,47.94 135.69,47.89
S$7404
  Bottom 0: 135.69,47.89 135.26,47.77
S$7405
  Bottom 0: 135.26,47.77 134.87,47.56
S$7406
  Bottom 0: 134.87,47.56 134.53,47.27
S$7407
  Bottom 0: 134.53,47.27 134.24,46.93
S$7408
  Bottom 0: 134.24,46.93 134.03,46.53
S$7409
  Bottom 0: 134.03,46.53 133.9,46.1
S$7410
  Bottom 0: 133.9,46.1 133.85,45.66
S$7411
  Bottom 0: 133.85,45.66 133.9,45.21
S$7412
  Bottom 0: 133.9,45.21 134.03,44.78
S$7413
  Bottom 0: 134.03,44.78 134.24,44.39
S$7414
  Bottom 0: 134.24,44.39 134.53,44.04
S$7415
  Bottom 0: 134.53,44.04 134.87,43.76
S$7416
  Bottom 0: 134.87,43.76 135.26,43.54
S$7417
  Bottom 0: 135.26,43.54 135.69,43.42
S$7418
  Bottom 0: 135.69,43.42 136.14,43.37
S$7419
  Bottom 0: 121.94,60.12 122.24,60.19
S$7420
  Bottom 0: 122.24,60.19 122.5,60.34
S$7421
  Bottom 0: 122.5,60.34 122.7,60.56
S$7422
  Bottom 0: 122.7,60.56 122.84,60.83
S$7423
  Bottom 0: 122.84,60.83 122.88,61.13
S$7424
  Bottom 0: 122.88,61.13 122.84,61.43
S$7425
  Bottom 0: 122.84,61.43 122.7,61.7
S$7426
  Bottom 0: 122.7,61.7 122.5,61.92
S$7427
  Bottom 0: 122.5,61.92 122.24,62.08
S$7428
  Bottom 0: 122.24,62.08 121.94,62.14
S$7429
  Bottom 0: 121.94,62.14 121.64,62.12
S$7430
  Bottom 0: 121.64,62.12 121.36,62.01
S$7431
  Bottom 0: 121.36,62.01 121.12,61.82
S$7432
  Bottom 0: 121.12,61.82 120.95,61.57
S$7433
  Bottom 0: 120.95,61.57 120.86,61.28
S$7434
  Bottom 0: 120.86,61.28 120.86,60.98
S$7435
  Bottom 0: 120.86,60.98 120.95,60.69
S$7436
  Bottom 0: 120.95,60.69 121.12,60.44
S$7437
  Bottom 0: 121.12,60.44 121.36,60.25
S$7438
  Bottom 0: 121.36,60.25 121.64,60.14
S$7439
  Bottom 0: 121.64,60.14 121.94,60.12
S$7440
  Bottom 0: 131.38,62.42 131.83,62.47
S$7441
  Bottom 0: 131.83,62.47 132.25,62.59
S$7442
  Bottom 0: 132.25,62.59 132.65,62.81
S$7443
  Bottom 0: 132.65,62.81 133,63.09
S$7444
  Bottom 0: 133,63.09 133.28,63.44
S$7445
  Bottom 0: 133.28,63.44 133.5,63.83
S$7446
  Bottom 0: 133.5,63.83 133.62,64.26
S$7447
  Bottom 0: 133.62,64.26 133.67,64.71
S$7448
  Bottom 0: 133.67,64.71 133.62,65.15
S$7449
  Bottom 0: 133.62,65.15 133.5,65.58
S$7450
  Bottom 0: 133.5,65.58 133.28,65.98
S$7451
  Bottom 0: 133.28,65.98 133,66.32
S$7452
  Bottom 0: 133,66.32 132.65,66.61
S$7453
  Bottom 0: 132.65,66.61 132.25,66.82
S$7454
  Bottom 0: 132.25,66.82 131.83,66.94
S$7455
  Bottom 0: 131.83,66.94 131.38,66.99
S$7456
  Bottom 0: 131.38,66.99 130.93,66.94
S$7457
  Bottom 0: 130.93,66.94 130.5,66.82
S$7458
  Bottom 0: 130.5,66.82 130.11,66.61
S$7459
  Bottom 0: 130.11,66.61 129.77,66.32
S$7460
  Bottom 0: 129.77,66.32 129.48,65.98
S$7461
  Bottom 0: 129.48,65.98 129.27,65.58
S$7462
  Bottom 0: 129.27,65.58 129.14,65.15
S$7463
  Bottom 0: 129.14,65.15 129.09,64.71
S$7464
  Bottom 0: 129.09,64.71 129.14,64.26
S$7465
  Bottom 0: 129.14,64.26 129.27,63.83
S$7466
  Bottom 0: 129.27,63.83 129.48,63.44
S$7467
  Bottom 0: 129.48,63.44 129.77,63.09
S$7468
  Bottom 0: 129.77,63.09 130.11,62.81
S$7469
  Bottom 0: 130.11,62.81 130.5,62.59
S$7470
  Bottom 0: 130.5,62.59 130.93,62.47
S$7471
  Bottom 0: 130.93,62.47 131.38,62.42
S$7472
  Bottom 0: 112.42,79.17 112.71,79.24
S$7473
  Bottom 0: 112.71,79.24 112.98,79.39
S$7474
  Bottom 0: 112.98,79.39 113.18,79.61
S$7475
  Bottom 0: 113.18,79.61 113.31,79.89
S$7476
  Bottom 0: 113.31,79.89 113.36,80.19
S$7477
  Bottom 0: 113.36,80.19 113.31,80.48
S$7478
  Bottom 0: 113.31,80.48 113.18,80.76
S$7479
  Bottom 0: 113.18,80.76 112.98,80.98
S$7480
  Bottom 0: 112.98,80.98 112.71,81.13
S$7481
  Bottom 0: 112.71,81.13 112.42,81.2
S$7482
  Bottom 0: 112.42,81.2 112.11,81.18
S$7483
  Bottom 0: 112.11,81.18 111.83,81.06
S$7484
  Bottom 0: 111.83,81.06 111.59,80.88
S$7485
  Bottom 0: 111.59,80.88 111.43,80.63
S$7486
  Bottom 0: 111.43,80.63 111.34,80.34
S$7487
  Bottom 0: 111.34,80.34 111.34,80.03
S$7488
  Bottom 0: 111.34,80.03 111.43,79.74
S$7489
  Bottom 0: 111.43,79.74 111.59,79.49
S$7490
  Bottom 0: 111.59,79.49 111.83,79.31
S$7491
  Bottom 0: 111.83,79.31 112.11,79.19
S$7492
  Bottom 0: 112.11,79.19 112.42,79.17
S$7493
  Bottom 0: 102.81,81.47 103.25,81.52
S$7494
  Bottom 0: 103.25,81.52 103.68,81.64
S$7495
  Bottom 0: 103.68,81.64 104.08,81.86
S$7496
  Bottom 0: 104.08,81.86 104.42,82.14
S$7497
  Bottom 0: 104.42,82.14 104.71,82.49
S$7498
  Bottom 0: 104.71,82.49 104.92,82.88
S$7499
  Bottom 0: 104.92,82.88 105.05,83.31
S$7500
  Bottom 0: 105.05,83.31 105.09,83.76
S$7501
  Bottom 0: 105.09,83.76 105.05,84.2
S$7502
  Bottom 0: 105.05,84.2 104.92,84.63
S$7503
  Bottom 0: 104.92,84.63 104.71,85.03
S$7504
  Bottom 0: 104.71,85.03 104.42,85.37
S$7505
  Bottom 0: 104.42,85.37 104.08,85.66
S$7506
  Bottom 0: 104.08,85.66 103.68,85.87
S$7507
  Bottom 0: 103.68,85.87 103.25,86
S$7508
  Bottom 0: 103.25,86 102.81,86.04
S$7509
  Bottom 0: 102.81,86.04 102.36,86
S$7510
  Bottom 0: 102.36,86 101.93,85.87
S$7511
  Bottom 0: 101.93,85.87 101.54,85.66
S$7512
  Bottom 0: 101.54,85.66 101.19,85.37
S$7513
  Bottom 0: 101.19,85.37 100.91,85.03
S$7514
  Bottom 0: 100.91,85.03 100.69,84.63
S$7515
  Bottom 0: 100.69,84.63 100.56,84.2
S$7516
  Bottom 0: 100.56,84.2 100.52,83.76
S$7517
  Bottom 0: 100.52,83.76 100.56,83.31
S$7518
  Bottom 0: 100.56,83.31 100.69,82.88
S$7519
  Bottom 0: 100.69,82.88 100.91,82.49
S$7520
  Bottom 0: 100.91,82.49 101.19,82.14
S$7521
  Bottom 0: 101.19,82.14 101.54,81.86
S$7522
  Bottom 0: 101.54,81.86 101.93,81.64
S$7523
  Bottom 0: 101.93,81.64 102.36,81.52
S$7524
  Bottom 0: 102.36,81.52 102.81,81.47
S$7525
  Bottom 0: 112.42,86.79 112.71,86.86
S$7526
  Bottom 0: 112.71,86.86 112.98,87.01
S$7527
  Bottom 0: 112.98,87.01 113.18,87.23
S$7528
  Bottom 0: 113.18,87.23 113.31,87.51
S$7529
  Bottom 0: 113.31,87.51 113.36,87.81
S$7530
  Bottom 0: 113.36,87.81 113.31,88.11
S$7531
  Bottom 0: 113.31,88.11 113.18,88.38
S$7532
  Bottom 0: 113.18,88.38 112.98,88.6
S$7533
  Bottom 0: 112.98,88.6 112.71,88.75
S$7534
  Bottom 0: 112.71,88.75 112.42,88.82
S$7535
  Bottom 0: 112.42,88.82 112.11,88.8
S$7536
  Bottom 0: 112.11,88.8 111.83,88.68
S$7537
  Bottom 0: 111.83,88.68 111.59,88.5
S$7538
  Bottom 0: 111.59,88.5 111.43,88.25
S$7539
  Bottom 0: 111.43,88.25 111.34,87.96
S$7540
  Bottom 0: 111.34,87.96 111.34,87.65
S$7541
  Bottom 0: 111.34,87.65 111.43,87.36
S$7542
  Bottom 0: 111.43,87.36 111.59,87.11
S$7543
  Bottom 0: 111.59,87.11 111.83,86.93
S$7544
  Bottom 0: 111.83,86.93 112.11,86.81
S$7545
  Bottom 0: 112.11,86.81 112.42,86.79
S$7546
  Bottom 0: 290.45,5.51 285.47,10.49
S$7547
  Bottom 0: 285.47,10.49 285.42,10.53
S$7548
  Bottom 0: 285.42,10.53 285.36,10.57
S$7549
  Bottom 0: 285.36,10.57 285.3,10.6
S$7550
  Bottom 0: 285.3,10.6 285.23,10.62
S$7551
  Bottom 0: 285.23,10.62 285.16,10.62
S$7552
  Bottom 0: 285.16,10.62 277.29,10.62
S$7553
  Bottom 0: 277.29,10.62 276.43,11.48
S$7554
  Bottom 0: 276.43,11.48 278.49,11.48
S$7555
  Bottom 0: 278.49,11.48 278.57,11.49
S$7556
  Bottom 0: 278.57,11.49 278.64,11.53
S$7557
  Bottom 0: 278.64,11.53 278.7,11.59
S$7558
  Bottom 0: 278.7,11.59 278.74,11.66
S$7559
  Bottom 0: 278.74,11.66 278.75,11.74
S$7560
  Bottom 0: 278.75,11.74 278.75,11.97
S$7561
  Bottom 0: 278.75,11.97 278.77,11.93
S$7562
  Bottom 0: 278.77,11.93 279.01,11.74
S$7563
  Bottom 0: 279.01,11.74 279.29,11.63
S$7564
  Bottom 0: 279.29,11.63 279.6,11.61
S$7565
  Bottom 0: 279.6,11.61 279.72,11.64
S$7566
  Bottom 0: 279.72,11.64 279.81,11.58
S$7567
  Bottom 0: 279.81,11.58 280.12,11.49
S$7568
  Bottom 0: 280.12,11.49 280.44,11.49
S$7569
  Bottom 0: 280.44,11.49 280.75,11.58
S$7570
  Bottom 0: 280.75,11.58 281.03,11.76
S$7571
  Bottom 0: 281.03,11.76 281.12,11.87
S$7572
  Bottom 0: 281.12,11.87 285.53,11.87
S$7573
  Bottom 0: 285.53,11.87 285.53,11.06
S$7574
  Bottom 0: 285.53,11.06 285.54,10.96
S$7575
  Bottom 0: 285.54,10.96 285.56,10.88
S$7576
  Bottom 0: 285.56,10.88 285.6,10.8
S$7577
  Bottom 0: 285.6,10.8 285.64,10.72
S$7578
  Bottom 0: 285.64,10.72 285.7,10.65
S$7579
  Bottom 0: 285.7,10.65 286.43,9.93
S$7580
  Bottom 0: 286.43,9.93 286.49,9.87
S$7581
  Bottom 0: 286.49,9.87 286.57,9.83
S$7582
  Bottom 0: 286.57,9.83 286.66,9.79
S$7583
  Bottom 0: 286.66,9.79 286.74,9.77
S$7584
  Bottom 0: 286.74,9.77 286.83,9.77
S$7585
  Bottom 0: 286.83,9.77 296.78,9.77
S$7586
  Bottom 0: 296.78,9.77 296.42,9.66
S$7587
  Bottom 0: 296.42,9.66 296.02,9.45
S$7588
  Bottom 0: 296.02,9.45 295.67,9.16
S$7589
  Bottom 0: 295.67,9.16 295.39,8.82
S$7590
  Bottom 0: 295.39,8.82 295.17,8.42
S$7591
  Bottom 0: 295.17,8.42 295.05,7.99
S$7592
  Bottom 0: 295.05,7.99 295,7.55
S$7593
  Bottom 0: 295,7.55 295.05,7.1
S$7594
  Bottom 0: 295.05,7.1 295.17,6.67
S$7595
  Bottom 0: 295.17,6.67 295.39,6.28
S$7596
  Bottom 0: 295.39,6.28 295.67,5.93
S$7597
  Bottom 0: 295.67,5.93 296.02,5.65
S$7598
  Bottom 0: 296.02,5.65 296.26,5.51
S$7599
  Bottom 0: 296.26,5.51 290.45,5.51
S$7600
  Bottom 0: 276.11,6.75 271.27,11.58
S$7601
  Bottom 0: 271.27,11.58 271.27,14.63
S$7602
  Bottom 0: 271.27,14.63 271.27,14.7
S$7603
  Bottom 0: 271.27,14.7 271.25,14.77
S$7604
  Bottom 0: 271.25,14.77 271.23,14.83
S$7605
  Bottom 0: 271.23,14.83 271.19,14.89
S$7606
  Bottom 0: 271.19,14.89 271.15,14.95
S$7607
  Bottom 0: 271.15,14.95 262.64,23.45
S$7608
  Bottom 0: 262.64,23.45 262.75,23.72
S$7609
  Bottom 0: 262.75,23.72 262.8,24.07
S$7610
  Bottom 0: 262.8,24.07 262.75,24.41
S$7611
  Bottom 0: 262.75,24.41 262.62,24.74
S$7612
  Bottom 0: 262.62,24.74 262.42,25.02
S$7613
  Bottom 0: 262.42,25.02 262.15,25.25
S$7614
  Bottom 0: 262.15,25.25 262.11,25.26
S$7615
  Bottom 0: 262.11,25.26 262.11,33.42
S$7616
  Bottom 0: 262.11,33.42 281.26,52.58
S$7617
  Bottom 0: 281.26,52.58 281.37,52.56
S$7618
  Bottom 0: 281.37,52.56 281.61,52.63
S$7619
  Bottom 0: 281.61,52.63 281.82,52.78
S$7620
  Bottom 0: 281.82,52.78 281.95,53
S$7621
  Bottom 0: 281.95,53 281.99,53.25
S$7622
  Bottom 0: 281.99,53.25 281.95,53.49
S$7623
  Bottom 0: 281.95,53.49 281.82,53.71
S$7624
  Bottom 0: 281.82,53.71 281.61,53.86
S$7625
  Bottom 0: 281.61,53.86 281.45,53.91
S$7626
  Bottom 0: 281.45,53.91 281.54,53.99
S$7627
  Bottom 0: 281.54,53.99 281.89,53.99
S$7628
  Bottom 0: 281.89,53.99 281.99,53.89
S$7629
  Bottom 0: 281.99,53.89 282.21,53.77
S$7630
  Bottom 0: 282.21,53.77 282.46,53.75
S$7631
  Bottom 0: 282.46,53.75 282.7,53.82
S$7632
  Bottom 0: 282.7,53.82 282.91,53.97
S$7633
  Bottom 0: 282.91,53.97 283.04,54.18
S$7634
  Bottom 0: 283.04,54.18 283.09,54.43
S$7635
  Bottom 0: 283.09,54.43 283.04,54.68
S$7636
  Bottom 0: 283.04,54.68 282.91,54.9
S$7637
  Bottom 0: 282.91,54.9 282.7,55.05
S$7638
  Bottom 0: 282.7,55.05 282.46,55.12
S$7639
  Bottom 0: 282.46,55.12 282.21,55.09
S$7640
  Bottom 0: 282.21,55.09 281.99,54.98
S$7641
  Bottom 0: 281.99,54.98 281.89,54.87
S$7642
  Bottom 0: 281.89,54.87 281.36,54.87
S$7643
  Bottom 0: 281.36,54.87 281.29,54.87
S$7644
  Bottom 0: 281.29,54.87 281.22,54.86
S$7645
  Bottom 0: 281.22,54.86 281.15,54.83
S$7646
  Bottom 0: 281.15,54.83 281.1,54.79
S$7647
  Bottom 0: 281.1,54.79 281.04,54.74
S$7648
  Bottom 0: 281.04,54.74 279.29,52.98
S$7649
  Bottom 0: 279.29,52.98 266.81,52.98
S$7650
  Bottom 0: 266.81,52.98 267,53.12
S$7651
  Bottom 0: 267,53.12 267.21,53.37
S$7652
  Bottom 0: 267.21,53.37 267.23,53.42
S$7653
  Bottom 0: 267.23,53.42 270.95,53.42
S$7654
  Bottom 0: 270.95,53.42 271.04,53.43
S$7655
  Bottom 0: 271.04,53.43 271.13,53.45
S$7656
  Bottom 0: 271.13,53.45 271.21,53.48
S$7657
  Bottom 0: 271.21,53.48 271.29,53.53
S$7658
  Bottom 0: 271.29,53.53 271.36,53.59
S$7659
  Bottom 0: 271.36,53.59 277.52,59.76
S$7660
  Bottom 0: 277.52,59.76 277.77,59.7
S$7661
  Bottom 0: 277.77,59.7 278.1,59.73
S$7662
  Bottom 0: 278.1,59.73 278.4,59.83
S$7663
  Bottom 0: 278.4,59.83 278.67,60.02
S$7664
  Bottom 0: 278.67,60.02 278.88,60.27
S$7665
  Bottom 0: 278.88,60.27 279.01,60.58
S$7666
  Bottom 0: 279.01,60.58 279.05,60.9
S$7667
  Bottom 0: 279.05,60.9 279.02,61.1
S$7668
  Bottom 0: 279.02,61.1 283.41,56.71
S$7669
  Bottom 0: 283.41,56.71 283.41,52.37
S$7670
  Bottom 0: 283.41,52.37 283.36,52.32
S$7671
  Bottom 0: 283.36,52.32 283.27,52.08
S$7672
  Bottom 0: 283.27,52.08 283.27,52.01
S$7673
  Bottom 0: 283.27,52.01 271.21,39.95
S$7674
  Bottom 0: 271.21,39.95 271.17,39.9
S$7675
  Bottom 0: 271.17,39.9 271.13,39.84
S$7676
  Bottom 0: 271.13,39.84 271.1,39.77
S$7677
